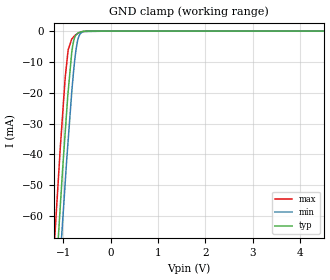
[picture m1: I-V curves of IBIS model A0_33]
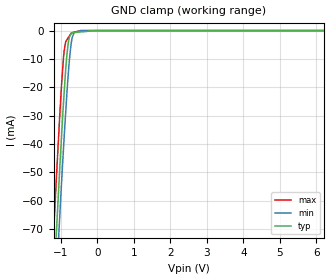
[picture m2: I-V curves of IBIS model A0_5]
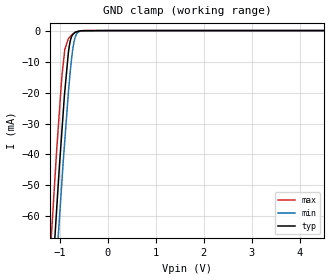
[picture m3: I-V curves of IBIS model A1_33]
|Texas Instruments Incorporated
|24-bit Analog-to-Digital Converter for Bridge Sensors
|ANALOG-TO-DIGITAL CONVERTER
| Marketing part#   Digital Voltage Range   Package-type   #pins
|INA226AIDGSR   2.7 V to 5.5 V   MSOP   10
[IBIS Ver]   4.0
[File name]   ina226.ibs
[File Rev]   1.0
|SimDE V3.0 201101 build 453
[Date]   06/16/2011
[Source]   Texas Instruments Incorporated.
   Analog-eLab, HPA
   12500 TI Blvd
   Dallas, TX -75243
   For Support e-mail: elab_ibis@list.ti.com
[Notes]   Revision History:
   1.0: 06/16/2011
   - Initial version of the model
   - Initial Model generated from simulations in TISPICED
   - Model names with a trailing _33 contains the model for
   3.3V (3V and 3.6V).
   _ Model names with trailing _5 contains
   the model for 5V (4.5V and 5.5V) operation.
   - Model not matched to measurements
   - C_comp although listed in numerical order of values are
   Obtained from varying PVT conditions. For PVT conditions
   for each specific value, refer the buffer description under
   respective [Model]. IBIS model user is responsible for using
   appropriate C_comp to simulate for Signal Integrity.
   - Combined Non-monotonic errors for SDA_33 and SDA_5 are minor
   and reflect SPICE transistor simulations
[Disclaimer]
  This model is designed as an aid for customers of Texas Instruments.
  TI and its licensors and suppliers make no warranties, either expressed
  or implied, with respect to this model, including the warranties of
  merchantability or fitness for a particular purpose.  The model is
  provided solely on an "as is" basis.  The entire risk as to its quality
  and performance is with the customer.
[Copyright] (C) Copyright 2011 Texas Instruments Incorporated.
   All rights reserved.
|   INA226
[Component]   ina226
[Manufacturer] TI
[Package]   | 10 MSOP - DSG package
| variable   typ   min   max
R_pkg  0.0472   0.0431   0.0588
L_pkg  1.5703nH  1.4822nH  1.8135nH
C_pkg  0.2483pF  0.2288pF  0.2613pF
|-------------------------PIN------------------------------------------------
[Pin] signal_name  model_name  R_pin  L_pin C_pin
1   A1   A1   0.04729  1.58129nH  0.22884pF
2   A0   A0   0.04342  1.49069nH  0.25510pF
3   Alert  ALERT   0.04310  1.48223nH  0.25511pF
4   SDA   SDA   0.04466  1.51585nH  0.25693pF
5   SCL   SCL   0.04770  1.58982nH  0.22875pF
6   Vs+   POWER   0.05311  1.69531nH  0.23513pF
7   GND   GND   0.04798  1.57681nH  0.26064pF
8   VBUS   TERM   0.04752  1.56504nH  0.26133pF
9   IN-   TERM   0.04543  1.52375nH  0.25891pF
10  IN+   TERM   0.05880  1.81346nH  0.24174pF
|   Model Selectors
[Model Selector]  A0
A0_33   3V digital input
A0_5   5V digital input
|NOTES   Model A0 split into two Models A0_33 and A0_5
|   to accommodate vast voltage range of 2.7V - 5.5V
|   A0_33 operates in voltage range of 3 - 3.3 - 3.6
|   A0_5 operates in voltage range of 4.5 - 5 - 5.5
|   The max pin frequency for Model A0 is 3.4MHz.Also the
|   voltage range and frequency is referenced with datasheet.
[Model Selector]  A1
A1_33   3V digital input
A1_5   5V digital input
|NOTES   Model A1 split into two Models A1_33 and A1_5
|   to accommodate vast voltage range of 2.7V - 5.5V
|   A1_33 operates in voltage range of 3 - 3.3 - 3.6
|   A1_5 operates in voltage range of 4.5 - 5 - 5.5
|   The max pin frequency for Model A1 is 3.4MHz.Also the
|   voltage range and frequency is referenced with datasheet.
[Model Selector]  SCL
SCL_33   3V digital input
SCL_5   5V digital input
|NOTES   Model SCL split into two Models SCL_33 and SCL_5
|   to accommodate vast voltage range of 2.7V - 5.5V
|   SCL_33 operates in voltage range of 3 - 3.3 - 3.6
|   SCL_5 operates in voltage range of 4.5 - 5 - 5.5
|   The max pin frequency for Model SCL is 3.4MHz.Also the
|   voltage range and frequency is referenced with datasheet.
[Model Selector]  ALERT
ALERT_33  3V digital open drain output
ALERT_5  5V digital open drain output
|NOTES   Model ALERT split into two Models ALERT_33 and ALERT_5
|   to accommodate vast voltage range of 2.7V - 5.5V
|   ALERT_33 operates in voltage range of 3 - 3.3 - 3.6
|   ALERT_5 operates in voltage range of 4.5 - 5 - 5.5
|   The max pin frequency for Model ALERT is 3.4MHz.Also the
|   voltage range and frequency is referenced with datasheet.
[Model Selector]  SDA
SDA_33  3V digital I/O open drain
SDA_5  5V digital I/O open drain
|NOTES   Model SDA split into two Models SDA_33 and SDA_5
|   to accommodate vast voltage range of 2.7V - 5.5V
|   SDA_33 operates in voltage range of 3 - 3.3 - 3.6
|   SDA_5 operates in voltage range of 4.5 - 5 - 5.5
|   The max pin frequency for Model SDA is 3.4MHz.Also the
|   voltage range and frequency is referenced with datasheet.
[Model Selector]  TERM
TERM_33  3V terminator
TERM_5  5V terminator
|   TERM Model
[Model] TERM_33
Model_type Terminator
C_comp   1e-20   1e-20   1e-20
| variable   typ   min   max
[Voltage Range]   3.3   3   3.6
|Ambient Temperature Range   27   85   -40
[Temperature Range]   30   88   -40
[Model] TERM_5
Model_type Terminator
C_comp   1e-20   1e-20   1e-20
| variable   typ   min   max
[Voltage Range]   5   4.5   5.5
|Ambient Temperature Range   27   85   -40
[Temperature Range]   30   88   -40
| Models and submodels in the file (12): A0_33 (Input), A0_5 (Input), A1_33 (Input), A1_5 (Input), SCL_33 (Input), SCL_5 (Input), ALERT_33 (Open_drain), ALERT_5 (Open_drain), SDA_33 (I/O_open_drain), SDA_5 (I/O_open_drain), TERM_33 (Terminator), TERM_5 (Terminator)
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|NOTES   Model TERM split into two Models TERM_33 and TERM_5
|   to accommodate vast voltage range of 2.7V - 5.5V
|   TERM_33 operates in voltage range of 3 - 3.3 - 3.6
|   TERM_5 operates in voltage range of 4.5 - 5 - 5.5
|   A0 input model
[Model]   A0_33
Model_type   Input
Vinl = 0.99   |min, GND -0.5 V
Vinh = 2.31   |max. V+ 6 V
|   typ   min   max
|   (nom PVT)   (Fast PVT)   (slow PVT)
C_comp   5.755E-13   5.651E-13   6.167E-13
| Where   nom PVT is Nominal Process, 3.3V, 25C
|   Fast PVT is Strong Process, 3.6V, -40C
|   Slow PVT is Weak Process, 3.0V, 85C
|C_comp - from L-C Tank method, L = 1nH, peak frequency
[Model Spec]
| variable   typ   min   max
Vinl   0.99   0.9   1.08
Vinh   2.31   2.1   2.52
|Vinl = 0.3 x V+, Vinh = 0.7 x V+
[Voltage Range]   3.3   3   3.6
|Ambient Temperature Range   27   85   -40
[Temperature Range]   30   88   -40
[Power Clamp Reference]   3.3   3   3.6
[GND Clamp Reference]   0   0   0
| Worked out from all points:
|   GND clamp passes 1 mA (typ) near -0.71 V on its own axis
[GND Clamp]
|   Voltage   I(typ)   I(min)   I(max)
-3.3V     -649.7mA   -656.5mA   -642.6mA
-1.178V   -84.67mA   -101.3mA   -66.35mA
-1.075V   -59.75mA   -76.11mA   -40.8mA
-1.064V   -56.98mA   -73.39mA   -37.96mA
-1.016V   -45.31mA   -62.27mA   -27.45mA
-958.6mV  -32.61mA   -48.92mA   -14.93mA
-897.4mV  -19.64mA   -35.49mA   -6.081mA
-803.9mV  -5.045mA   -16.67mA   -2.273mA
-731.9mV  -1.28mA    -6.1mA     -1.161mA
-683.6mV  -535.5uA   -2.309mA   -623.7uA
-571.3mV  -63.02uA   -161.1uA   -123.6uA
6.59V     0A         0A         0A
[POWER Clamp]
|   SCR cell for ESD function. Effects occurr above VDD x 2
|   Voltage   I(typ)   I(min)   I(max)
-3.3V     0A         0A         0A
0V        0A         0A         0A
6.6V      0A         0A         0A
[Model]   A0_5
Model_type   Input
Vinl = 1.5   |min, GND -0.5 V
Vinh = 3.5   |max. V+ 6 V
|   typ   min   max
|   (nom PVT)   (Fast PVT)   (slow PVT)
C_comp   5.650E-13   5.547E-13   5.971E-13
| Where   nom PVT is  Nominal Process, 3.3V, 25C
|   Fast PVT is Strong Process, 3.6V, -40C
|   Slow PVT is Weak Process, 3.0V, 85C
|C_comp - from L-C Tank method, L = 1nH, peak frequency
[Model Spec]
| variable   typ   min   max
Vinl   1.5   1.35   1.65
Vinh   3.5   3.15   3.85
|Vinl = 0.3 x V+, Vinh = 0.7 x V+
[Voltage Range]   5   4.5   5.5
|Ambient Temperature Range   27   85   -40
[Temperature Range]   30   88   -40
[Power Clamp Reference]   5   4.5   5.5
[GND Clamp Reference]   0   0   0
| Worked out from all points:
|   GND clamp passes 1 mA (typ) near -0.72 V on its own axis
[GND Clamp]
|   Voltage   I(typ)   I(min)   I(max)
-5V       -1.111A    -1.111A    -1.112A
-1.23V    -97.87mA   -113.9mA   -79.44mA
-1.131V   -73.49mA   -90.01mA   -54.25mA
-1.04V    -51.13mA   -68.06mA   -32.3mA
-980.8mV  -37.34mA   -53.79mA   -19.29mA
-920.4mV  -24.21mA   -40.24mA   -8.706mA
-862.7mV  -13.06mA   -28.08mA   -3.821mA
-797mV    -4.411mA   -15.56mA   -2.529mA
-707mV    -797.3uA   -3.787mA   -833.3uA
-624.4mV  -696.4uA   -567.2uA   -533.2uA
-434.8mV  -464.7uA   -3.534uA   -3.641uA
9.985V    0A         0A         0A
[POWER Clamp]
|   SCR cell for ESD function. Effects occurr above VDD x 2
|   Voltage   I(typ)   I(min)   I(max)
-5V       0A         0A         0A
0V        0A         0A         0A
10V       0A         0A         0A
|   A1 input model
[Model]   A1_33
Model_type   Input
Vinl = 0.99   |min, GND -0.5 V
Vinh = 2.31   |max. V+ 6 V
|   typ   min   max
|   (nom PVT)   (Fast PVT)   (slow PVT)
C_comp   5.836E-13   5.547E-13   6.340E-13
| Where   nom PVT is  Nominal Process, 3.3V, 25C
|   Fast PVT is Strong Process, 3.6V, -40C
|   Slow PVT is Weak Process, 3.0V, 85C
|C_comp - from L-C Tank method, L = 1nH, peak frequency
[Model Spec]
| variable   typ   min   max
Vinl   0.99   0.9   1.08
Vinh   2.31   2.1   2.52
|Vinl = 0.3 x V+, Vinh = 0.7 x V+
[Voltage Range]   3.3   3   3.6
|Ambient Temperature Range   27   85   -40
[Temperature Range]   30   88   -40
[Power Clamp Reference]   3.3   3   3.6
[GND Clamp Reference]   0   0   0
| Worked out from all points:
|   GND clamp passes 1 mA (typ) near -0.71 V on its own axis
[GND Clamp]
|   Voltage   I(typ)   I(min)   I(max)
-3.3V     -649.7mA   -656.5mA   -642.6mA
-1.178V   -84.67mA   -101.3mA   -66.35mA
-1.073V   -59.17mA   -75.54mA   -40.21mA
-1.064V   -56.98mA   -73.4mA    -37.96mA
-1.016V   -45.31mA   -62.27mA   -27.45mA
-958.6mV  -32.61mA   -48.9mA    -14.93mA
-897.4mV  -19.64mA   -35.5mA    -6.08mA
-803.9mV  -5.045mA   -16.68mA   -2.273mA
-735.4mV  -1.334mA   -6.489mA   -1.2mA
-683.6mV  -535.5uA   -2.3mA     -623.7uA
-573.6mV  -64.07uA   -170.3uA   -127.6uA
6.59V     0A         0A         0A
[POWER Clamp]
|   SCR cell for ESD function. Effects occurr above VDD x 2
|   Voltage   I(typ)   I(min)   I(max)
-3.3V     0A         0A         0A
0V        0A         0A         0A
6.6V      0A         0A         0A
